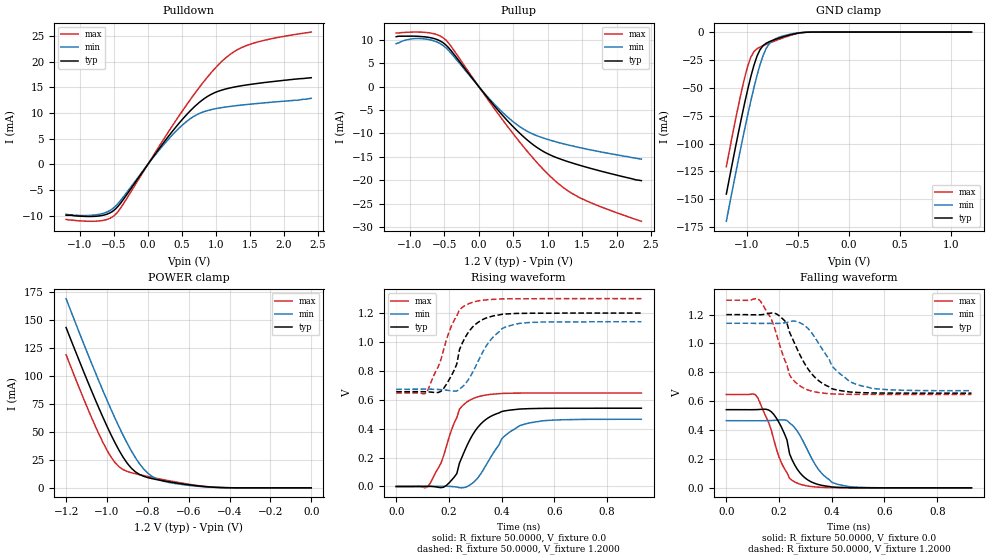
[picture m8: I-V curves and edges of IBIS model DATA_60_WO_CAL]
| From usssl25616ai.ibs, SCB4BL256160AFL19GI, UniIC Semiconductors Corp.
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|   Model DATA_60_WO_CAL
[Model]  DATA_60_WO_CAL
Model_type I/O
Polarity   Non-Inverting
Enable   Active-High
Vinl =   0.3800V
Vinh =   0.8200V
Vmeas =  0.6000V
Cref =   5.0000pF
Rref =   50.0000
Vref =   0.6000V
C_comp   1.7430pF   1.7110pF   1.7640pF
[Temperature Range]   25.0000   85.0000   -40.0000
[Voltage Range]   1.2000V   1.1400V   1.3000V
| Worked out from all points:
|   slope of the pulldown table from 0 to 0.18 V, typ, clamps not added: 54.2 ohm
|   slope of the pullup table from 0 to 0.18 V, typ, clamps not added: 54.6 ohm
|   GND clamp passes 1 mA (typ) near -0.50 V on its own axis
|   POWER clamp passes 1 mA (typ) near -0.51 V on its own axis
|   rising waveform, R_fixture 50.0000, V_fixture 0.0: 20-80 % time 88.7ps typ, 104ps min, 76.6ps max; typ from 0 V to 0.542 V
|   rising waveform, R_fixture 50.0000, V_fixture 1.2000: 20-80 % time 75.5ps typ, 92.4ps min, 81.4ps max; typ from 0.656 V to 1.2 V
|   falling waveform, R_fixture 50.0000, V_fixture 0.0: 20-80 % time 72.3ps typ, 89.7ps min, 77.3ps max; typ from 0.542 V to 0 V
|   falling waveform, R_fixture 50.0000, V_fixture 1.2000: 20-80 % time 98.8ps typ, 115ps min, 71ps max; typ from 1.2 V to 0.656 V
[Pulldown]
|Voltage   I(typ)   I(min)   I(max)
-1.2V     -9.9mA     -9.7mA     -10.7mA
-760mV    -10.09mA   -9.816mA   -11.05mA
-600mV    -9.689mA   -9.267mA   -10.72mA
-480mV    -8.742mA   -8.201mA   -9.813mA
-360mV    -6.833mA   -6.334mA   -7.71mA
200mV     3.678mA    3.335mA    4.233mA
520mV     8.97mA     7.816mA    10.66mA
840mV     12.94mA    10.35mA    16.44mA
1.2V      14.89mA    11.29mA    21.36mA
1.36V     15.3mA     11.55mA    22.66mA
1.6V      15.77mA    11.87mA    23.82mA
2.4V      16.9mA     12.9mA     25.8mA
[Pullup]
|Voltage   I(typ)   I(min)   I(max)
-1.2V     10.7mA     9.2mA      11.5mA
-1V       10.81mA    10.17mA    11.66mA
-840mV    10.73mA    10.29mA    11.67mA
-680mV    10.41mA    9.918mA    11.42mA
-520mV    9.417mA    8.82mA     10.48mA
-400mV    7.656mA    7.103mA    8.572mA
320mV     -5.719mA   -5.15mA    -6.596mA
600mV     -10.04mA   -8.607mA   -11.97mA
840mV     -12.96mA   -10.47mA   -16.16mA
1.12V     -15.13mA   -11.8mA    -20.3mA
1.4V      -16.53mA   -12.82mA   -23.23mA
2.36V     -20.1mA    -15.5mA    -28.79mA
[GND_clamp]
|Voltage   I(typ)   I(min)   I(max)
-1.2V     -145.3mA   -169.7mA   -120.8mA
-1.11V    -103.1mA   -127.3mA   -78.51mA
-1.05V    -76.2mA    -100.1mA   -52.43mA
-990mV    -51.2mA    -74mA      -30.39mA
-960mV    -39.9mA    -61.63mA   -22.48mA
-900mV    -21.67mA   -39mA      -15mA
-870mV    -15.78mA   -29.25mA   -13.45mA
-810mV    -10.04mA   -14.72mA   -11.07mA
-750mV    -7.557mA   -7.71mA    -8.865mA
-600mV    -3.111mA   -2.463mA   -3.804mA
-420mV    -215.4uA   -156.1uA   -235uA
1.2V      1.597nA    5.589nA    1.463nA
[POWER_clamp]
|Voltage   I(typ)   I(min)   I(max)
-1.2V     143mA      168.8mA    118.7mA
-1.06V    79.88mA    104.3mA    56.26mA
-1.02V    63.08mA    86.79mA    40.63mA
-980mV    47.32mA    69.97mA    27.48mA
-940mV    33.2mA     54.05mA    18.67mA
-880mV    17.43mA    32.78mA    13.45mA
-840mV    11.87mA    21.34mA    11.69mA
-800mV    9.133mA    13.1mA     10.12mA
-720mV    6.135mA    5.731mA    7.166mA
-560mV    1.838mA    1.456mA    2.161mA
-420mV    156.9uA    132.7uA    153uA
0V        1.597nA    1.927nA    2.16nA
[Ramp]
| variable   typ   min   max
dV/dt_r  0.3250/88.8406p   0.2791/0.1064n   0.3881/77.1250p
dV/dt_f  0.3264/93.6061p   0.2801/0.1158n   0.3917/75.3477p
R_load = 50.0000
[Rising Waveform]
R_fixture= 50.0000
V_fixture= 0.0
V_fixture_min= 0.0
V_fixture_max= 0.0
|time   V(typ)   V(min)   V(max)
0s        0V         0V         0V
120ps     1.169mV    197.5uV    -632.8uV
170ps     -8.318mV   1.072mV    162.2mV
220ps     64.7mV     -1.731mV   439.1mV
240ps     162.2mV    -8.679mV   534.8mV
300ps     386.3mV    39.95mV    614.6mV
400ps     518.7mV    329.4mV    643.6mV
470ps     536mV      421.8mV    646.2mV
590ps     541mV      458.7mV    646.8mV
930ps     541.6mV    465.1mV    646.8mV
[Rising Waveform]
R_fixture= 50.0000
V_fixture= 1.2000
V_fixture_min= 1.1400
V_fixture_max= 1.3000
|time   V(typ)   V(min)   V(max)
0s        656mV      673mV      647.1mV
110ps     655.3mV    673.6mV    642.9mV
170ps     658.9mV    669.9mV    879.8mV
220ps     805mV      659.8mV    1.15V
230ps     848.4mV    660.5mV    1.18V
240ps     946.5mV    673.8mV    1.223V
280ps     1.082V     757.7mV    1.268V
350ps     1.171V     995.1mV    1.293V
420ps     1.194V     1.107V     1.298V
930ps     1.2V       1.14V      1.3V
[Falling Waveform]
R_fixture= 50.0000
V_fixture= 0.0
V_fixture_min= 0.0
V_fixture_max= 0.0
|time   V(typ)   V(min)   V(max)
0s        541.6mV    465.1mV    646.8mV
110ps     541.7mV    464.6mV    645.6mV
160ps     539.8mV    465.7mV    454.9mV
180ps     508.7mV    467.3mV    334.5mV
230ps     331.8mV    466.8mV    105.2mV
240ps     234.8mV    449.2mV    65.31mV
270ps     126.6mV    390.9mV    31.85mV
350ps     22.47mV    126.3mV    4.671mV
410ps     4.87mV     31.39mV    868.9uV
930ps     0V         0V         0V
[Falling Waveform]
R_fixture= 50.0000
V_fixture= 1.2000
V_fixture_min= 1.1400
V_fixture_max= 1.3000
|time   V(typ)   V(min)   V(max)
0s        1.2V       1.14V      1.3V
130ps     1.199V     1.139V     1.292V
170ps     1.211V     1.139V     1.171V
230ps     1.14V      1.145V     848.6mV
250ps     1.037V     1.155V     756mV
310ps     823.2mV    1.104V     677.8mV
400ps     687mV      846.1mV    650.7mV
480ps     662.5mV    726.3mV    647.6mV
600ps     656.7mV    681.5mV    647.1mV
930ps     656mV      673.1mV    647.1mV
